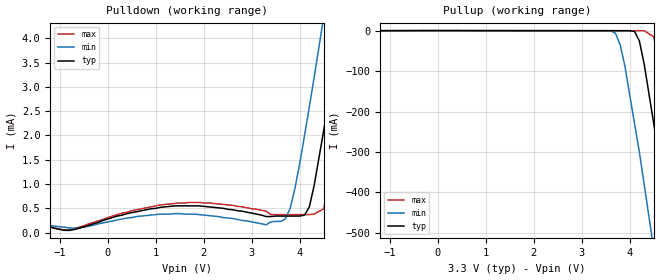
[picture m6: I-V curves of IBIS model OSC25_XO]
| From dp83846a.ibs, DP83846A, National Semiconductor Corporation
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|   Model OSC25_XO
[Model]   OSC25_XO
Model_type   Output
Polarity   Inverting
Enable   Active-High
Vmeas =   1.50V
Cref =  10.00pF
Rref = 100.00k
C_comp   5.00pF   5.00pF   5.00pF
[Temperature Range]   25.00   0.14k   0.000
[Voltage Range]   3.30V   3.00V   3.60V
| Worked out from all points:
|   slope of the pulldown table from 0 to 0.495 V, typ, clamps not added: 3.84 kohm
|   slope of the pullup table from 0 to 0.495 V, typ, clamps not added: 5.7 kohm
[Pulldown]
| voltage   I(typ)   I(min)   I(max)
-3.3V     240uA      210uA      270uA
-800mV    44.54uA    95.09uA    59.2uA
1.7V      550uA      380uA      620uA
3.6V      340uA      230uA      370uA
3.9V      340uA      910uA      370uA
4.1V      360uA      2mA        370uA
4.3V      970uA      3.2mA      380uA
4.5V      2.11mA     4.45mA     490uA
4.9V      4.63mA     7.03mA     2.62mA
5.1V      5.93mA     8.34mA     3.89mA
5.3V      7.26mA     9.66mA     5.18mA
6.6V      16.11mA    18.46mA    13.95mA
[Pullup]
| voltage   I(typ)   I(min)   I(max)
-3.3V     -460uA     -400uA     -500uA
3.6V      -280uA     -810uA     -310uA
3.8V      -290uA     -34.77mA   -310uA
3.9V      -290uA     -88.81mA   -310uA
4.1V      -2.22mA    -230mA     -320uA
4.3V      -82.47mA   -380mA     -330uA
4.5V      -230mA     -540mA     -15.28mA
4.7V      -390mA     -700mA     -140mA
4.9V      -550mA     -870mA     -290mA
5.1V      -720mA     -1.03A     -450mA
5.3V      -880mA     -1.2A      -620mA
6.6V      -1.98A     -2.29A     -1.71A
[Ramp]
| variable   typ   min   max
dV/dt_r   1.17/12.10n   0.95/14.11n   1.30/11.38n
dV/dt_f   1.35/8.89n   1.02/12.07n   1.49/8.28n
R_load = 10.00k
| End [Model] OSC25_XO
